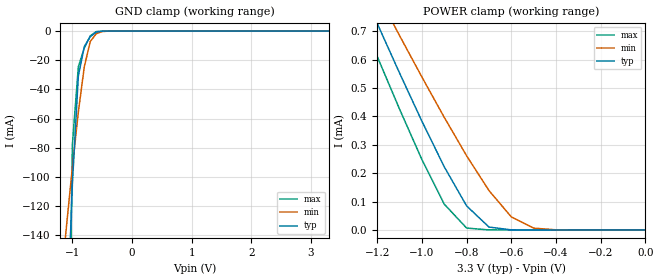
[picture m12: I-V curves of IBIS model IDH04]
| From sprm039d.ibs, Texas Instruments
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[Model]   IDH04
Model_type   Input
Polarity   Non-Inverting
| signals   A, Y
Vinl = 0.8V
Vinh = 2.0V
|   typ   min   max
C_comp   1.6130p   1.5354p   1.7989p
|   typ   min   max
[Temperature Range]   25   -40   125
|   typ   min   max
[Voltage Range]   3.30V   3.00V   3.60V
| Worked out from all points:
|   GND clamp passes 1 mA (typ) near -0.61 V on its own axis
|   POWER clamp passes 1 mA (typ) near -1.35 V on its own axis
[GND_clamp]
|   Voltage   I(typ)   I(min)   I(max)
-3.3V     -3.217A    -1.141A    -10.79A
-1.2V     -338.8mA   -177.1mA   -773.3mA
-1.1V     -215.6mA   -134.5mA   -364.4mA
-1V       -105mA     -93.53mA   -78.21mA
-900mV    -30.86mA   -55.63mA   -24.55mA
-800mV    -10.62mA   -24.48mA   -11.59mA
-700mV    -3.849mA   -7.151mA   -3.3mA
-600mV    -739.7uA   -1.805mA   -366.3uA
-500mV    -67.29uA   -326.4uA   -17.03uA
-400mV    -3.755uA   -40.31uA   -379.9nA
3.3V      133.2pA    31.66nA    133.2pA
[POWER_clamp]
|   Voltage   I(typ)   I(min)   I(max)
-3.3V     4.6mA      4.102mA    4.747mA
-1.3V     905.1uA    983.5uA    800.7uA
-1.2V     727.5uA    833.2uA    611.3uA
-1.1V     552.9uA    684.6uA    425.8uA
-1V       383.1uA    538.7uA    248.1uA
-900mV    222.6uA    396.7uA    91.01uA
-800mV    84.8uA     261.3uA    6.786uA
-700mV    10.3uA     138.9uA    73.81nA
-600mV    329.7nA    46.05uA    977pA
-500mV    8.438nA    6.46uA     177.6pA
-400mV    355.3pA    466.5nA    222pA
0V        1pA        1pA        1pA
